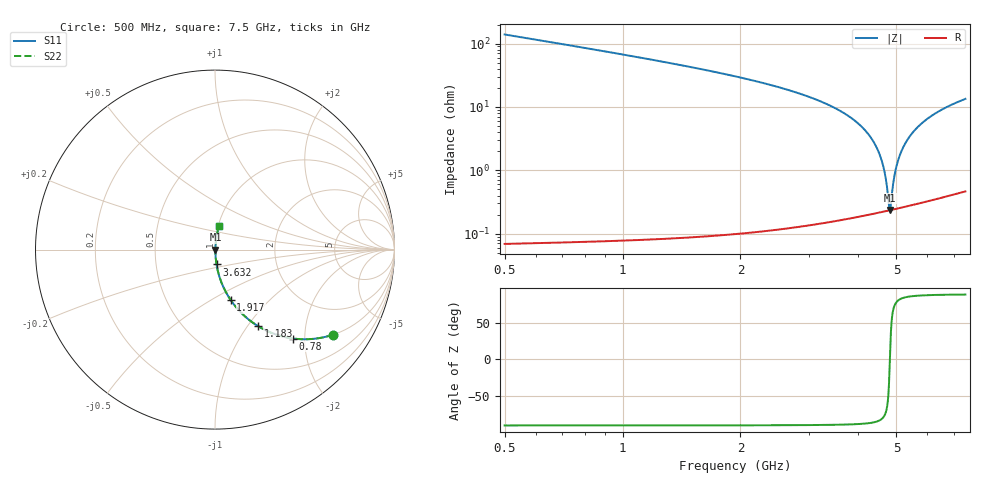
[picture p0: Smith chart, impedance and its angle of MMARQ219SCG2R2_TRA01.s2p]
! MMARQ219SCG2R2_TRA01  S-PARAMETER MODEL  ( General Type )
! Model Generated by TAIYO YUDEN Corporation (http://www.ty-top.com)
! Version 1.0
! TAIYO YUDEN Control No. 160201
! Copyright(c) 2016 TAIYO YUDEN CO.,LTD. All Rights Reserved.
! Product Description (link to TY-COMPAS)
! https://ds.yuden.co.jp/TYCOMPAS/or/detail?pn=MMARQ219SCG2R2BTRA01&u=M
! Products Name : Multilayer Ceramic Capacitors
! Characteristics :
!  Capacitance : 2.2 pF , Rated Voltage : 250V , TCC : CG / C0G
!  Case Size : 2.0 x 1.25 / 0.079 x 0.049 [mm/inch] , Thickness : 0.85 / 0.033 [mm/inch]
!  (Conditions: Temperature = 25 degC , DC Bias Current/Voltage = 0A / 0V)
! External Node Assignments :
!  1  o---| |---o  2
! GND o---------o GND
! Frequency Range : 500MHz  -  7500MHz  [ 401 STEP ]
# MHz S RI R 50
! Freq[MHz].  S11 Real  S11 Imag  S21 Real  S21 Imag  S12 Real  S12 Imag  S22 Real  S22 Imag
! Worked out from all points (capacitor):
!   401 points, 500 MHz to 7.5 GHz, reference 50 ohm
!   read as one part in series: C = 2.26 pF near 535 MHz
!   lowest |Z| = 237 mohm at 4.805 GHz (marker M1)
!   series resonance near 4.812 GHz, so ESL is about 480 pH
!   S11 on the Smith chart (normalised r, x): 500 MHz: 1.00, -2.79; 780 MHz: 1.00, -1.76; 1.183 GHz: 1.00, -1.12; 1.917 GHz: 1.00, -0.62; 3.632 GHz: 1.00, -0.17; 7.5 GHz: 1.01, +0.27
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500  0.6598 -0.4735  0.3402 0.4735  0.3402 0.4735  0.6598 -0.4735
780  0.4358 -0.4954  0.5642 0.4954  0.5642 0.4954  0.4358 -0.4954
1182.5  0.2387 -0.4255  0.7613 0.4255  0.7613 0.4255  0.2387 -0.4255
1672.5  0.1211 -0.325  0.8789 0.325  0.8789 0.325  0.1211 -0.325
1917.5  0.0878 -0.2814  0.9122 0.2814  0.9122 0.2814  0.0878 -0.2814
2845  0.0264 -0.1565  0.9736 0.1565  0.9736 0.1565  0.0264 -0.1565
3632.5  0.00851 -0.0825  0.9915 0.0825  0.9915 0.0825  0.00851 -0.0825
4000  0.00477 -0.054  0.9952 0.054  0.9952 0.054  0.00477 -0.054
4315  0.00303 -0.0318  0.997 0.0318  0.997 0.0318  0.00303 -0.0318
4542.5  0.00244 -0.0168  0.9976 0.0168  0.9976 0.0168  0.00244 -0.0168
4665  0.00232 -0.00904  0.9977 0.00904  0.9977 0.00904  0.00232 -0.00904
4717.5  0.00231 -0.00578  0.9977 0.00578  0.9977 0.00578  0.00231 -0.00578
4787.5  0.00232 -0.00149  0.9977 0.00149  0.9977 0.00149  0.00232 -0.00149
4805  0.00233 -0.000426  0.9977 0.000426  0.9977 0.000426  0.00233 -0.000426
4840  0.00236 0.00169  0.9976 -0.00169  0.9976 -0.00169  0.00236 0.00169
4910  0.00244 0.00587  0.9976 -0.00587  0.9976 -0.00587  0.00244 0.00587
4980  0.00255 0.00999  0.9975 -0.00999  0.9975 -0.00999  0.00255 0.00999
5172.5  0.00303 0.021  0.997 -0.021  0.997 -0.021  0.00303 0.021
5365  0.00373 0.0317  0.9963 -0.0317  0.9963 -0.0317  0.00373 0.0317
5627.5  0.00501 0.0456  0.995 -0.0456  0.995 -0.0456  0.00501 0.0456
6345  0.0101 0.0808  0.9899 -0.0808  0.9899 -0.0808  0.0101 0.0808
7500  0.022 0.1305  0.978 -0.1305  0.978 -0.1305  0.022 0.1305
